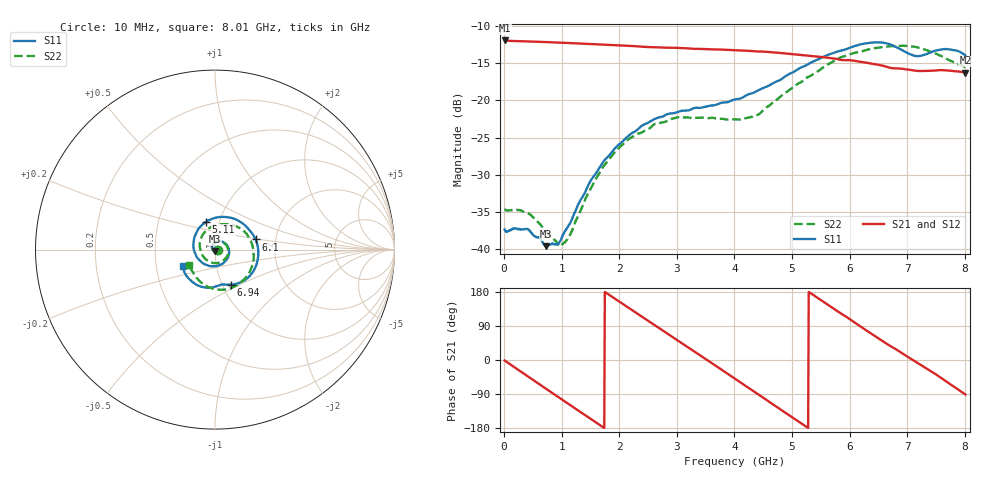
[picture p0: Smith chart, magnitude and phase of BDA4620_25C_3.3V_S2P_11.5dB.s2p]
!Agilent Technologies,E5071B,MY42404982,A.09.10
!Date: Wed May 06 08:50:54 2026
!Data & Calibration Information:
!Freq	S11:SOLT2(ON)	S21:SOLT2(ON)	S12:SOLT2(ON)	S22:SOLT2(ON)
# Hz S RI R 50
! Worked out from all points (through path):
!   801 points, 10 MHz to 8.01 GHz, reference 50 ohm
!   highest |S21| = -11.93 dB at 10 MHz (marker M1); lowest = -16.3 dB at 8.01 GHz (marker M2)
!   group delay of S21, straight-line fit = 281 ps
!   lowest |S11| = -39.6 dB at 720 MHz (marker M3), VSWR 1.02, Z = 50 - j1.05 ohm
!   |S11| at or under -10 dB: start of sweep to end of sweep
!   |S22| runs from -39.5 to -12.6 dB; largest |S21 - S12| = 0.001
!   S11 on the Smith chart (normalised r, x): 10 MHz: 1.03, -0.00; 5.11 GHz: 0.86, +0.27; 6.1 GHz: 1.57, +0.19; 6.94 GHz: 1.10, -0.45; 8.01 GHz: 0.69, -0.13
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1e7  0.0136 -0.000905  0.253 -0.00546  0.2534 -0.00557  0.0186 -0.00111
4e8  0.0108 -0.00843  0.1858 -0.1663  0.186 -0.1667  0.0145 -0.00978
7.2e8  0.00056 -0.0105  0.0643 -0.2384  0.0643 -0.2387  0.00358 -0.013
1.01e9  -0.0114 -0.00415  -0.062 -0.2362  -0.0623 -0.2366  -0.00873 -0.00639
1.35e9  -0.0166 0.0146  -0.1836 -0.1563  -0.1837 -0.1563  -0.0148 0.0119
1.66e9  -0.00624 0.035  -0.2351 -0.0364  -0.2353 -0.0363  -0.00702 0.0319
1.93e9  0.014 0.0459  -0.2228 0.0753  -0.223 0.0756  0.011 0.0437
2.32e9  0.0513 0.0381  -0.121 0.1968  -0.1213 0.1971  0.0448 0.0395
2.68e9  0.0766 0.00501  0.018 0.2268  0.0182 0.2271  0.0685 0.015
3.39e9  0.037 -0.081  0.2158 0.0529  0.2162 0.0527  0.0468 -0.0604
4.01e9  -0.0677 -0.0755  0.1416 -0.1654  0.1417 -0.1659  -0.0424 -0.0616
4.52e9  -0.1206 0.0198  -0.043 -0.2082  -0.0432 -0.2087  -0.0852 0.019
5.11e9  -0.0512 0.1545  -0.1932 -0.0624  -0.1937 -0.0623  -0.0145 0.1293
5.35e9  0.0175 0.1807  -0.1973 0.0224  -0.1974 0.0225  0.0446 0.1418
5.69e9  0.1277 0.1625  -0.1451 0.1265  -0.1452 0.1269  0.1329 0.1224
6.1e9  0.2261 0.0564  -0.0242 0.1828  -0.024 0.183  0.2079 0.0253
6.39e9  0.2375 -0.0595  0.0657 0.1639  0.0657 0.164  0.2143 -0.062
6.68e9  0.1755 -0.1635  0.1288 0.1057  0.1293 0.1059  0.179 -0.1466
6.94e9  0.0904 -0.195  0.1573 0.042  0.1577 0.0419  0.1171 -0.2017
7.19e9  0.0366 -0.1949  0.1561 -0.0234  0.1565 -0.0236  0.0355 -0.2242
7.58e9  -0.07 -0.2082  0.1102 -0.1158  0.1107 -0.116  -0.0764 -0.1845
8.01e9  -0.1788 -0.0923  -0.00251 -0.1536  -0.00246 -0.154  -0.143 -0.0855
